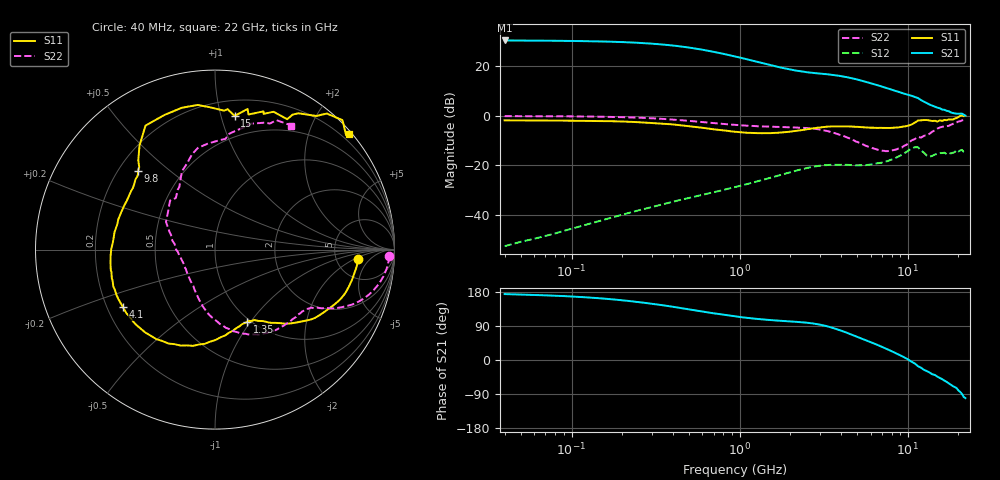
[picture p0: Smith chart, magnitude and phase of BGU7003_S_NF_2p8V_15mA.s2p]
!	Filename:	P:\Prog\Test\Noise\ATS_data\Testdata_Net\BGU7002	BGU7003	RN20082092\BGU7003_B1_high	freq_bias	loop_2.88V13.6mA_D.s2p
!	Date/Time:	Tue	16-Sep-08	9:24:57
!	BGU7003_B1_high	freq_bias	loop
!	bias	mode	1:00	Vout=	2.88	"V,"	Iout=13.5700	"mA,"	Vin=	5.676	"V,"	Iin=	1.3815	mA
!	Date/time	Mon	Aug	11	5:02:53	2008
!	Device	data	file	deembeded	for	feedlines	and	parallel
!	Original	file:	\BGU7002	BGU7003	RN20082092\BGU7003_B1_high	freq_bias	loop_2.88V13.6mA_R.s2p
!	Feed-files:	PR029V01_high	"frequency_140808_Feed1.s2p,"	PR029V01_high	frequency_140808_Feed2.s2p
!	Parallel-file:	PR029V01_high	frequency_140808_Par.s2p
#	MHz	S	MA	R	50
!	Freq-MHz	S11-mag	S11-arg	S21-mag	S21-arg	S12-mag	S12-arg	S22-mag	S22-arg
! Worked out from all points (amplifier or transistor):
!   160 points, 40 MHz to 22 GHz, reference 50 ohm
!   highest |S21| = 30.2 dB at 40 MHz (marker M1)
!   |S21| within 3 dB of that: start of sweep to 515.3 MHz
!   unconditionally stable (mu >= 1): nowhere
!   at 300 MHz: K = 0.37, MSG = 32.9 dB, |S12| = -36.8 dB
!   at 2.25 GHz: K = 0.63, MSG = 19.9 dB, |S12| = -21.9 dB
!   at 22 GHz: K = -0.02, MSG = 7.5 dB, |S12| = -15.0 dB
!   lowest NFmin = 0.71 dB at 400 MHz
!   S11 on the Smith chart (normalised r, x): 40 MHz: 8.28, -2.48; 1.35 GHz: 0.96, -0.96; 4.1 GHz: 0.27, -0.27; 9.8 GHz: 0.28, +0.39; 15 GHz: 0.32, +1.11; 22 GHz: 0.06, +2.70
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40  0.8005 -3.9  32.5 174.0  0.00234 59.1  0.9722 -2.2
70  0.7944 -7.0  32.07 170.6  0.00377 69.1  0.9678 -4.4
120  0.7821 -12.2  31.47 165.6  0.00623 73.8  0.9566 -7.7
160  0.772 -16.2  30.87 161.6  0.00817 74.5  0.9429 -10.2
210  0.7544 -20.9  29.97 156.6  0.01052 74.1  0.9229 -13.1
270  0.7226 -26.1  28.7 151.1  0.01317 73.1  0.8959 -16.1
330  0.6933 -31.1  27.32 146.0  0.01566 71.9  0.8663 -18.7
420  0.6508 -37.1  25.25 139.0  0.01911 70.2  0.819 -22.1
550  0.586 -44.7  22.23 130.6  0.0236 68.6  0.7596 -25.3
700  0.5274 -50.7  19.18 123.2  0.02849 67.2  0.7039 -27.5
950  0.4702 -57.8  15.32 114.9  0.03655 65.8  0.648 -30.1
1100  0.4499 -60.8  13.58 111.3  0.0414 64.9  0.6245 -31.2
1350  0.4396 -66.1  11.44 107.3  0.04984 63.0  0.6044 -33.6
1950  0.4691 -80.2  8.582 102.1  0.07046 55.7  0.5804 -42.0
2700  0.5498 -102.8  7.262 96.7  0.09256 43.0  0.5479 -58.0
4100  0.6046 -148.1  6.132 75.8  0.1012 23.9  0.3892 -90.3
5600  0.5783 179.7  4.792 52.7  0.1 20.5  0.2478 -117.8
7800  0.5614 151.1  3.422 25.6  0.1254 21.9  0.1937 -161.7
9800  0.6123 134.6  2.682 4.2  0.1841 13.3  0.2567 162.1
11500  0.7921 119.3  2.245 -16.4  0.2293 -20.0  0.3707 132.5
15000  0.7529 81.6  1.438 -44.1  0.1684 -29.3  0.5475 103.4
22000  0.9845 40.7  0.9924 -100.6  0.1773 -80.4  0.8054 58.5
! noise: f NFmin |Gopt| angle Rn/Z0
400  0.715  0.132  14.95  0.117
1000  0.811  0.139  31.58  0.129
1500  0.891  0.146  45.44  0.134
1700  0.923  0.15  50.99  0.136
2200  1.003  0.158  64.85  0.136
3000  1.132  0.174  87.03  0.132
4400  1.357  0.208  125.8  0.116
5800  1.581  0.25  164.7  0.101
8000  1.935  0.334  -152.8  0.112
1.2e+04  2.577  0.537  -111  0.404
